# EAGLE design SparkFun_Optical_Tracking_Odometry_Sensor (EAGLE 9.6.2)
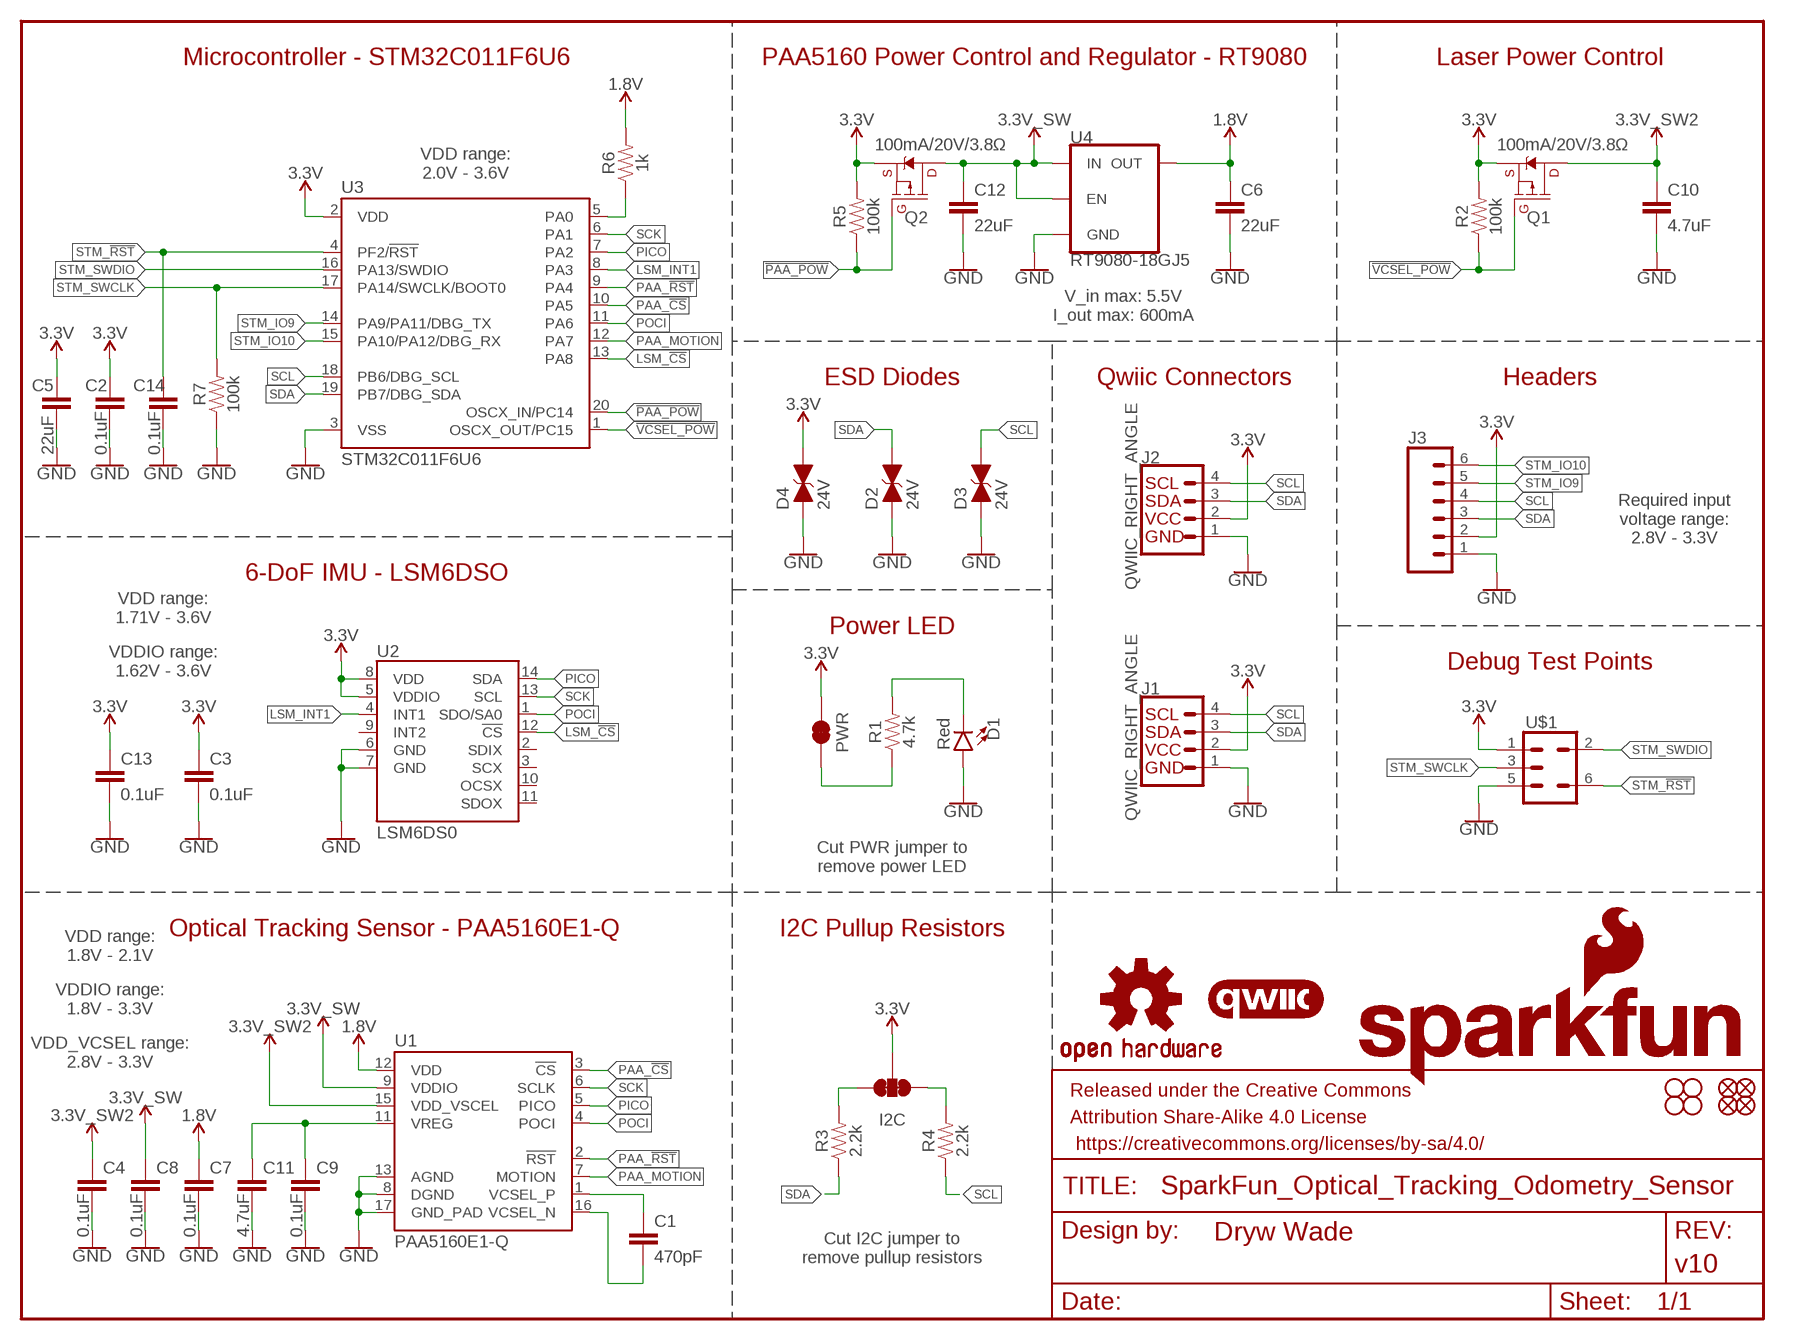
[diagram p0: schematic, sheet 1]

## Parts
C1  470pF  470PF-0603-50V-5%  [0603]
C2  0.1uF  0.1UF-0603-25V-(+80/-20%)  [0603]
C3  0.1uF  0.1UF-0603-25V-(+80/-20%)  [0603]
C4  0.1uF  0.1UF-0603-25V-(+80/-20%)  [0603]
C5  22uF  22UF-0603-6.3V-20%  [0603]
C6  22uF  22UF-0603-6.3V-20%  [0603]
C7  0.1uF  0.1UF-0603-25V-(+80/-20%)  [0603]
C8  0.1uF  0.1UF-0603-25V-(+80/-20%)  [0603]
C9  0.1uF  0.1UF-0603-25V-(+80/-20%)  [0603]
C10  4.7uF  4.7UF-0603-6.3V-(10%)  [0603]
C11  4.7uF  4.7UF-0603-6.3V-(10%)  [0603]
C12  22uF  22UF-0603-6.3V-20%  [0603]
C13  0.1uF  0.1UF-0603-25V-(+80/-20%)  [0603]
C14  0.1uF  0.1UF-0603-25V-(+80/-20%)  [0603]
D1  Red  LED-RED_0603-KB  [LED-0603]
D2  24V  DIODE_TVS  [0603]
D3  24V  DIODE_TVS  [0603]
D4  24V  DIODE_TVS  [0603]
FD1  FIDUCIAL1X2  [FIDUCIAL-1X2]
FD2  FIDUCIAL1X2  [FIDUCIAL-1X2]
FD3  FIDUCIAL1X2  [FIDUCIAL-1X2]
FD4  FIDUCIAL1X2  [FIDUCIAL-1X2]
FRAME1  FRAME-LETTER  [CREATIVE_COMMONS]
H1  STAND-OFF  [STAND-OFF]
H2  STAND-OFF  [STAND-OFF]
H3  STAND-OFF  [STAND-OFF]
H4  STAND-OFF  [STAND-OFF]
I2C  JUMPER-SMT_3_2-NC_TRACE_SILK  [SMT-JUMPER_3_2-NC_TRACE_SILK]
J1  QWIIC_RIGHT_ANGLE  QWIIC_CONNECTORJS-1MM  [JST04_1MM_RA]
J2  QWIIC_RIGHT_ANGLE  QWIIC_CONNECTORJS-1MM  [JST04_1MM_RA]
J3  CONN_06NO_SILK_NO_POP  [1X06_NO_SILK]
LOGO1  OSHW-LOGOS  [OSHW-LOGO-S]
LOGO2  QWIIC_LOGO_5MM  [QWIIC_5MM]
LOGO3  SFE_LOGO_NAME_FLAME.1_INCH  [SFE_LOGO_NAME_FLAME_.1]
PWR  JUMPER-SMT_2_NC_TRACE_SILK  [SMT-JUMPER_2_NC_TRACE_SILK]
Q1  100mA/20V/3.8Ω  MOSFET_PCH-RE1C001ZPTL  [SOT-416FL]
Q2  100mA/20V/3.8Ω  MOSFET_PCH-RE1C001ZPTL  [SOT-416FL]
R1  4.7k  4.7KOHM-0603-1/10W-1%  [0603]
R2  100k  100KOHM-0603-1/10W-1%  [0603]
R3  2.2k  2.2KOHM-0603-1/10W-1%  [0603]
R4  2.2k  2.2KOHM-0603-1/10W-1%  [0603]
R5  100k  100KOHM-0603-1/10W-1%  [0603]
R6  1k  1KOHM-0603-1/10W-1%  [0603]
R7  100k  100KOHM-0603-1/10W-1%  [0603]
U1  PAA5160E1-Q  [PAA5160E1-Q]
U2  LSM6DS0  LSM6DSO  [LGA14L]
U3  STM32C011F6U6  [STM32C011F6U6]
U4  RT9080-18GJ5  V_REG_RT9080-18GJ5  [SOT23-5]
U$1  SWD-5PIN  [PAD_05_03X2_TP_NO4]

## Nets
1.8V: C6.1 C7.1 R6.2 U1.12(VDD) U4.5(OUT)
3.3V: C2.1 C3.1 C5.1 C13.1 D4.2(C) I2C.2 J1.2 J2.2 J3.2 PWR.2 Q1.2(S) Q2.2(S) R2.2 R5.2 U2.5(VDDIO) U2.8(VDD) U3.2(VDD) U$1.1
3.3V_SW: C8.1 C12.1 Q2.3(D) U1.9(VDDIO) U4.1(IN) U4.3(EN)
3.3V_SW2: C4.1 C10.1 Q1.3(D) U1.15(VDD_VSCEL)
!PAA_POW!: Q2.1(G) R5.1 U3.20(OSCX_IN/PC14)
!VCSEL_POW!: Q1.1(G) R2.1 U3.1(OSCX_OUT/PC15)
GND: C2.2 C3.2 C4.2 C5.2 C6.2 C7.2 C8.2 C9.2 C10.2 C11.2 C12.2 C13.2 C14.2 D1.A D2.1(A) D3.1(A) D4.1(A) J1.1 J2.1 J3.1 R7.1 U1.8(DGND) U1.13(AGND) U1.17(GND_PAD) U2.6(GND) U2.7(GND) U3.3(VSS) U4.2(GND) U$1.5
LSM_!CS!: U2.12(!CS!) U3.13(PA8)
LSM_INT1: U2.4(INT1) U3.8(PA3)
N$1: PWR.1 R1.1
N$2: D1.C R1.2
N$3: C1.1 U1.1(VCSEL_P)
N$4: C1.2 U1.16(VCSEL_N)
N$5: I2C.3 R3.2
N$6: I2C.1 R4.2
N$7: C9.1 C11.1 U1.11(VREG)
N$8: R6.1 U3.5(PA0)
PAA_!CS!: U1.3(!CS!) U3.10(PA5)
PAA_!RST!: U1.2(!RST!) U3.9(PA4)
PAA_MOTION: U1.7(MOTION) U3.12(PA7)
PICO: U1.5(PICO) U2.14(SDA) U3.7(PA2)
POCI: U1.4(POCI) U2.1(SDO/SA0) U3.11(PA6)
SCK: U1.6(SCLK) U2.13(SCL) U3.6(PA1)
SCL: D3.2(C) J1.4 J2.4 J3.4 R4.1 U3.18(PB6/DBG_SCL)
SDA: D2.2(C) J1.3 J2.3 J3.3 R3.1 U3.19(PB7/DBG_SDA)
STM_!RST!: C14.1 U3.4(PF2/!RST!) U$1.6
STM_IO9: J3.5 U3.14(PA9/PA11/DBG_TX)
STM_IO10: J3.6 U3.15(PA10/PA12/DBG_RX)
STM_SWCLK: R7.2 U3.17(PA14/SWCLK/BOOT0) U$1.3
STM_SWDIO: U3.16(PA13/SWDIO) U$1.2
Unconnected: U2.2(SDIX) U2.3(SCX) U2.9(INT2) U2.10(OCSX) U2.11(SDOX)

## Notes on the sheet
- Microcontroller - STM32C011F6U6 | PAA5160 Power Control and Regulator - RT9080 | Laser Power Control
- VDD range:
  2.0V - 3.6V
- V_in max: 5.5V
  I_out max: 600mA
- ESD Diodes | Qwiic Connectors | Headers
- Required input
  voltage range:
  2.8V - 3.3V
- 6-DoF IMU - LSM6DSO
- VDD range:
  1.71V - 3.6V
- Power LED
- VDDIO range:
  1.62V - 3.6V
- Debug Test Points
- Cut PWR jumper to
  remove power LED
- Optical Tracking Sensor - PAA5160E1-Q | I2C Pullup Resistors
- VDD range:
  1.8V - 2.1V
- VDDIO range:
  1.8V - 3.3V
- VDD_VCSEL range:
  2.8V - 3.3V
- Cut I2C jumper to
  remove pullup resistors

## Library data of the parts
C1 = SparkFun-Capacitors:470PF: 470pF ceramic capacitors; PROD_ID: CAP-07884
C2-C4 C7-C9 C13 C14 = SparkFun-Capacitors:0.1UF: 0.1µF ceramic capacitors; PROD_ID: CAP-00810
C5 C6 C12 = SparkFun-Capacitors:22UF: 22µF ceramic capacitors; PROD_ID: CAP-14464
C10 C11 = SparkFun-Capacitors:4.7UF: 4.7µF ceramic capacitors; PROD_ID: CAP-08280
D1 = SparkFun-LED:LED-RED: Red SMD LED; PROD_ID: DIO-17976
D2-D4 = SparkFun-DiscreteSemi:DIODE_TVS; PROD_ID: DIO-14502
FD1-FD4 = SparkFun-Aesthetics:FIDUCIAL: Fiducial Alignment Points
FRAME1 = SparkFun-Aesthetics:FRAME-LETTER: Schematic Frame - Letter; DESIGNER: Dryw Wade; REV: v10
H1-H4 = SparkFun-Hardware:STAND-OFF: Stand Off
I2C = SparkFun-Jumpers:JUMPER-SMT_3_2-NC_TRACE: Normally closed trace jumper (2 of 2 connections) This jumper has a trace between all three pads so they are normally closed (NC). Use a razor knife to open the connection(s). For best results follow the IPC guidelines for cutting traces: Cutout at least 0.063 mm (0.005 in). Remove all loose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
J1 J2 = SparkFun-Connectors:QWIIC_CONNECTOR: SparkFun I2C Standard Qwiic Connector An SMD 1mm pitch JST connector makes it easy and quick (get it? Qwiic?) to connect I2C devices to each other. The Qwiic system enables fast and solderless connection between popular platforms and various sensors and actuators. We carry 200mm, 100mm, 50mm, and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; PROD_ID: CONN-13694
J3 = SparkFun-Connectors:CONN_06: Multi connection point. Often used as Generic Header-pin footprint for 0.1 inch spaced/style header connections On any of the 0.1 inch spaced packages, you can populate with these: Break Away Headers - Straight (PRT-00116) Break Away Male Headers - Right Angle (PRT-00553) Female Headers (PRT-00115)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
LOGO1 = SparkFun-Aesthetics:OSHW-LOGO: Open-Source Hardware (OSHW) Logo
LOGO2 = SparkFun-Aesthetics:QWIIC_LOGO: Qwiic Logos for placement on schematic and PCB. The 5.5mm silk logo is best for placing next to Qwiic connector.
LOGO3 = SparkFun-Aesthetics:SFE_LOGO_NAME_FLAME: SparkFun Font Logo w/ Flame
PWR = SparkFun-Jumpers:JUMPER-SMT_2_NC_TRACE: Normally closed trace jumper
Q1 Q2 = SparkFun-DiscreteSemi:MOSFET_PCH: P-channel MOSFETs Voltage controlled devices that allow control of high current outputs. SparkFun Products: SparkFun ESP32 Thing SparkFun ESP8266 Thing SparkFun Pi Servo HAT V2 DMG2305UX-7 (20V/4.2A/SOT23-3); PROD_ID: TRANS-15421
R1 = SparkFun-Resistors:4.7KOHM: 4.7kΩ resistor; PROD_ID: RES-07857
R2 R5 R7 = SparkFun-Resistors:100KOHM: 100kΩ resistor; PROD_ID: RES-07828
R3 R4 = SparkFun-Resistors:2.2KOHM: 2.2kΩ resistor; PROD_ID: RES-08272
R6 = SparkFun-Resistors:1KOHM: 1kΩ resistor; PROD_ID: RES-07856
U1 = Optical_Tracking_Odometry_Sensor:PAA5160E1-Q; PROD_ID: IC-21320
U2 = SparkFun-Sensors:LSM6DSO: The LSM6DSO is a system-in-package featuring a high-performance 3-axis digital accelerometer and 3-axis digital gyroscope.; PROD_ID: IC-15837
U3 = Optical_Tracking_Odometry_Sensor:STM32C011F6U6; PROD_ID: IC-21321
U4 = SparkFun-IC-Power:V_REG_RT9080-18GJ5: RT9080-18GJ5 Low-Dropout Linear Regulator The RT9080 is a low-dropout (LDO) voltage regulators with enable function that operates from 1.2V to 5.5V. It provides up to 600mA of output current and offers low-power operation in miniaturized packaging. The features of low quiescent current as low as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; PROD_ID: VREG-21045
U$1 = SparkFun-Connectors:SWD-5PIN: 5-pin SWD connector Test-point based header for SWD. Pin 1 - PWR Pin 2 - SWDIO Pin 3 - SWCLK Pin 4 - NC Pin 5 - GND Pin 6 - RESET

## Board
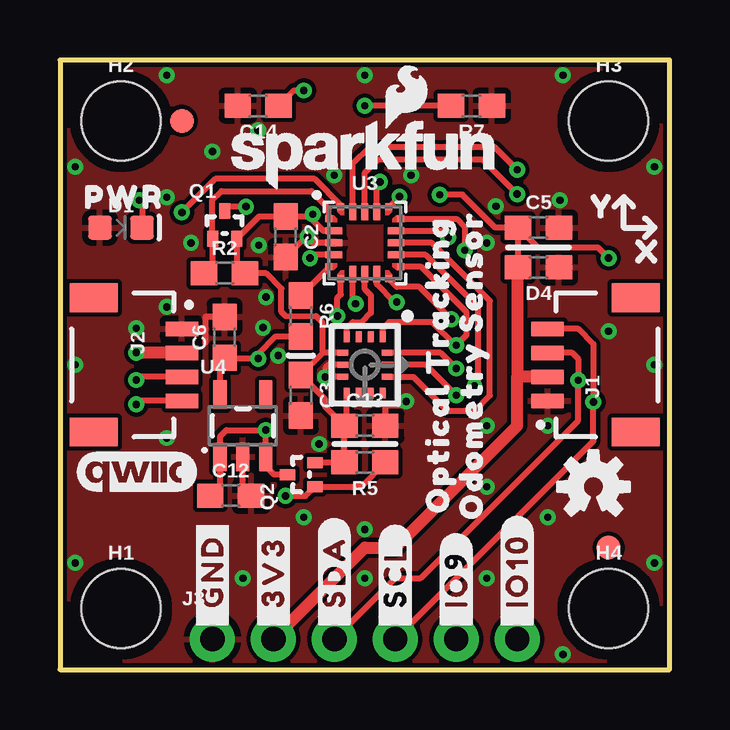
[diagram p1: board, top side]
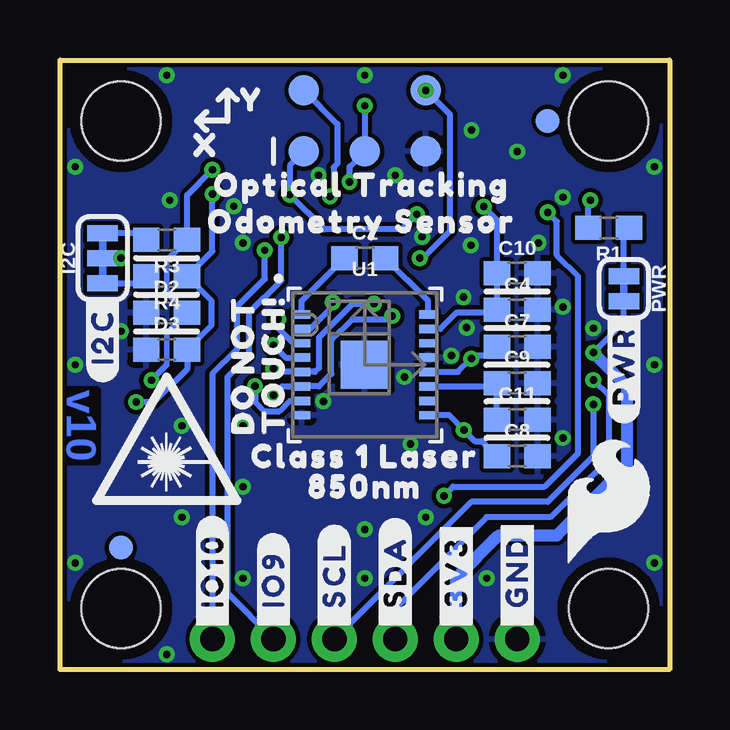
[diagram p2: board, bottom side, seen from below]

Size 25.4 x 25.4 mm. Coordinates in mm from the lower left corner, seen from the top.
Outline: 0,0 25.4,0 25.4,25.4 0,25.4 0,0
Copper layers (1*16): Top 0.035mm / dielectric 1.5mm / Bottom 0.035mm
Design rules "SparkFun-2-Layer-General-JLCPCB": minimum track width 7mil, minimum drill 0.3mm, track to track 7mil, track to pad 7mil, pad to pad 7mil, via to via 7mil, smd to smd 7mil, copper to edge 7mil, drill to drill 7mil, minimum pad ring 7mil, minimum via ring 7mil, stop-mask expansion 3mil, vias tented up to drill 25mil, thermal gap 10mil
tRestrict: area 6.7,16.1 to 7,16.3

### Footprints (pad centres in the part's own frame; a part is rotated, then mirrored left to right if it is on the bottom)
0603 = smd 1.1 x 1: 1 -0.85,0; 2 0.85,0
LED-0603 = smd 1 x 1: A -0.877,0; C 0.877,0
FIDUCIAL-1X2 = smd 1 x 1: 1 0,0
STAND-OFF = hole 3.302: 0,0
SMT-JUMPER_3_2-NC_TRACE_SILK = smd 0.66 x 1.27: 1 -1.041,0; 2 0,0; 3 1.041,0
JST04_1MM_RA = smd 0.6 x 1.35: 1 -1.5,0; 2 -0.5,0; 3 0.5,0; 4 1.5,0 | smd 1.2 x 2: NC1 2.8,-3.675; NC2 -2.8,-3.675
1X06_NO_SILK = drill 1.016 pad 1.88: 1 0,0; 2 2.54,0; 3 5.08,0; 4 7.62,0; 5 10.16,0; 6 12.7,0
SMT-JUMPER_2_NC_TRACE_SILK = smd 0.66 x 1.27: 1 -0.521,0; 2 0.521,0
SOT-416FL = smd 0.46 x 0.65: 1 -0.5,-1.1; 2 0.5,-1.1; 3 0,0.05
PAA5160E1-Q = smd 0.73 x 0.35: 1 -2.635,2.1; 2 -2.635,1.5; 3 -2.635,0.9; 4 -2.635,0.3; 5 -2.635,-0.3; 6 -2.635,-0.9; 7 -2.635,-1.5; 8 -2.635,-2.1; 9 2.635,-2.1; 10 2.635,-1.5; 11 2.635,-0.9; 12 2.635,-0.3; 13 2.635,0.3; 14 2.635,0.9; 15 2.635,1.5; 16 2.635,2.1 | smd 2 x 2: 17 0,0
LGA14L = smd 0.45 x 0.25: 1 -1.175,0.75; 2 -1.175,0.25; 3 -1.175,-0.25; 4 -1.175,-0.75; 8 1.175,-0.75; 9 1.175,-0.25; 10 1.175,0.25; 11 1.175,0.75 | smd 0.25 x 0.45: 5 -0.5,-0.925; 6 0,-0.925; 7 0.5,-0.925; 12 0.5,0.925; 13 0,0.925; 14 -0.5,0.925
STM32C011F6U6 = smd 0.3 x 0.3: 1 -1.5,1; 5 -1.5,-1; 6 -1,-1.5; 10 1,-1.5; 11 1.5,-1; 15 1.5,1; 16 1,1.5; 20 -1,1.5 | smd 0.7 x 0.3: 2 -1.3,0.5; 3 -1.3,0; 4 -1.3,-0.5; 12 1.3,-0.5; 13 1.3,0; 14 1.3,0.5 | smd 0.3 x 0.7: 7 -0.5,-1.3; 8 0,-1.3; 9 0.5,-1.3; 17 0.5,1.3; 18 0,1.3; 19 -0.5,1.3
SOT23-5 = smd 0.55 x 1.2: 1 -0.95,-1.3; 2 0,-1.3; 3 0.95,-1.3; 4 0.95,1.3; 5 -0.95,1.3
PAD_05_03X2_TP_NO4 = smd 1.27 x 1.27: 1 -2.54,-1.27; 2 -2.54,1.27; 3 0,-1.27; 5 2.54,-1.27; 6 2.54,1.27

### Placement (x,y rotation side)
C1  12.7,17.14 0 bottom
C2  9.4,18.03 270 top
C3  10.03,11.43 270 top
C4  6.35,14.99 0 bottom
C5  19.94,18.41 0 top
C6  6.86,13.84 90 top
C7  6.35,13.46 0 bottom
C8  6.35,8.89 0 bottom
C9  6.35,11.94 0 bottom
C10  6.35,16.51 0 bottom
C11  6.35,10.41 0 bottom
C12  7.11,7.24 0 top
C13  12.7,10.16 0 top
C14  8.26,23.5 180 top
D1  2.54,18.41 0 top
D2  20.95,14.86 0 bottom
D3  20.95,13.34 0 bottom
D4  19.94,16.76 180 top
FD1  5.08,22.86 0 bottom
FD2  5.08,22.86 0 top
FD3  22.86,5.08 0 bottom
FD4  22.86,5.08 0 top
FRAME1  not placed on the board
H1  2.54,2.54 0 top
H2  2.54,22.86 0 top
H3  22.86,22.86 0 top
H4  22.86,2.54 0 top
I2C  23.62,17.14 90 bottom
J1  20.32,12.7 90 top
J2  5.08,12.7 270 top
J3  6.35,1.27 0 top
LOGO1  22.23,7.62 0 top
LOGO2  3.17,8.26 0 top
LOGO3  12.7,21.46 0 top
PWR  1.91,15.88 270 bottom
Q1  6.86,19.05 0 top
Q2  9.53,8.13 90 top
R1  2.54,18.41 180 bottom
R2  6.86,16.51 0 top
R3  20.95,17.91 180 bottom
R4  20.95,16.38 180 bottom
R5  12.7,8.64 180 top
R6  10.03,14.73 270 top
R7  17.14,23.5 180 top
U1  12.7,12.7 0 bottom
U2  12.7,12.7 270 top
U3  12.7,17.78 0 top
U4  7.62,10.16 0 top
U$1  12.7,22.86 0 bottom
U$2  [#_GND#0]  6.35,1.52 90 top
U$3  [#_3V3#0]  8.89,1.52 90 top
U$4  [#_SDA#0]  11.43,1.52 90 top
U$5  [#_SCL#0]  13.97,1.52 90 top
U$6  [CLASS_1_LASER0]  12.7,8.89 0 bottom
U$7  [#_IO10#0]  19.05,1.52 90 top
U$8  [#_GND#0]  6.35,1.52 90 bottom
U$9  [#_3V3#0]  8.89,1.52 90 bottom
U$10  [#_SDA#0]  11.43,1.52 90 bottom
U$11  [#_SCL#0]  13.97,1.52 90 bottom
U$12  [#_IO9#0]  16.51,1.52 90 top
U$14  [OPTICAL_TRACKING0]  12.83,20.19 0 bottom
U$15  [ODOMETRY_SENSOR0]  12.83,18.67 0 bottom
U$16  [OPTICAL_TRACKING0]  15.75,12.7 90 top
U$17  [ODOMETRY_SENSOR0]  17.14,12.7 90 top
U$18  [X0]  24.51,17.4 0 top
U$20  [#PWR#0]  1.91,14.99 90 bottom
U$21  [TOUCH##0]  16.51,12.7 90 bottom
U$22  [DO_NOT0]  17.78,12.7 90 bottom
U$23  [#_IO10#0]  19.05,1.52 90 bottom
U$24  [SFE_LOGO_FLAME_.2]  2.54,6.99 0 bottom
U$25  [PWR0]  2.67,19.68 0 top
U$26  [#I2C#0]  23.62,15.75 90 bottom
U$27  [ORDERING_INSTRUCTIONS]  not placed on the board
U$28  [850NM0]  12.7,7.62 0 bottom
U$29  [Y0]  22.61,19.3 0 top
U$30  [X0]  19.3,21.84 0 bottom
U$31  [Y0]  17.4,23.75 0 bottom
U$32  [#_IO9#0]  16.51,1.52 90 bottom

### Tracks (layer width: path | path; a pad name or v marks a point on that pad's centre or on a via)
1.8V  (via drill 0.3)
  Top 0.254: U4.5 6.67,12.8 C6.1 6.89,12.96 v8.26,12.96 8.26,13.15 8.99,13.88 R6.2
  Bottom 0.254: C7.1 7.56,13.11 8.11,13.11 v8.26,12.96 8.82,12.4 U1.12
3.3V  (via drill 0.3)
  Top 0.229: 10.67,14.73 9.4,14.73
  Top 0.254: C13.1 11.95,10.26 U2.8 | 10.94,13.19 C3.1 11.05,11.26 11.05,10.96 C13.1 | 10.94,13.19 10.95,13.2 U2.5 | U3.2 10.97,18.28 10.53,18.72 v10.53,18.97 10.44,18.88 C2.1 8.29,18.88 Q1.2 7.36,16.86 R2.2 8.59,16.51 9.22,15.88 9.22,14.91 9.4,14.73 | 10.94,13.19 10.94,14.45 10.92,14.47 10.92,14.48 10.67,14.73 | Q2.2 10.63,8.64 R5.2 C13.1 | 19.05,16.73 D4.2 C5.1 | v22.86,17.14 22.42,17.59 19.91,17.59 C5.1 | C5.1 18.14,18.41 16.77,19.79 v15.82,19.79
  Top 0.508: J2.2 3.18,13.2 v3.17,13.21 | J3.2 12.7,5.08 13.97,5.08 19.05,10.16 19.05,12.2 | J1.2 19.05,12.2 | 19.05,16.73 19.05,12.2
  Bottom 0.254: v10.53,18.97 11.17,18.34 14.38,18.34 v15.82,19.79 15.82,21.01 U$1.1 | I2C.2 v22.86,17.14 | v3.17,13.21 1.91,14.48 PWR.2
  Bottom 0.508: J3.2 8.89,3.81 7.11,5.59 4.7,5.59 1.78,8.51 1.78,11.81 v3.17,13.21
3.3V_SW  (via drill 0.3)
  Top 0.254: C12.1 6.67,7.65 U4.1 6.67,9.72 6.93,9.98 v8.57,9.98 U4.3 8.57,8.48 8.92,8.13 Q2.3
  Bottom 0.254: C8.1 7.83,9.53 8.12,9.53 v8.57,9.98 9.19,10.6 U1.9
3.3V_SW2  (via drill 0.3)
  Top 0.254: Q1.3 7.05,19.29 v7.75,19.29
  Bottom 0.254: U1.15 9.55,14.2 8.87,14.88 7.3,14.88 C4.1 C10.1 7.2,18.74 v7.75,19.29
!PAA_POW!  (via drill 0.3)
  Top 0.254: U3.20 11.7,19.36 10.61,20.45 6.48,20.45 v5.08,19.05 | R5.1 12.54,7.63 Q2.1 10.24,7.24 v9.4,7.24
  Bottom 0.254: v5.08,19.05 4.7,18.67 4.7,17.27 3.81,16.38 3.81,9.02 5.21,7.62 9.02,7.62 v9.4,7.24
!VCSEL_POW!
  Top 0.254: U3.1 11.2,19.21 10.47,19.94 6.73,19.94 6.32,19.53 6.32,17.98 Q1.1 6.36,16.86 R2.1
GND  (via drill 0.3)
  Top 0.254: U2.7 v11.06,12.2 | v11.06,12.2 v11.05,12.19 | U2.6 11.18,12.7 11.06,12.57 v11.06,12.2 | U3.3 10.51,17.78 10.38,17.91 10.12,17.91 C2.2 | C12.2 7.62,7.58 U4.2 | C6.2 6.05,14.69 6.05,14.22 | 6.05,14.22 6.05,13.63 | J2.1 6.03,14.2 6.05,14.22 | v14.43,11.18 14.25,10.99 13.55,10.99 C13.2
  other vias: 9.09,13.08 4.45,15.11 4.45,9.65 3.17,14.22 8.59,15.52 8.46,14.25 10.79,9.4 5.46,17.78 8.28,17.68 20.32,10.16 17.78,7.62 17.78,10.16 17.78,3.81 20.32,6.35 17.78,17.78 22.86,14.1 18.16,19.3 20.83,19.56 11.43,20.6 4.45,19.68 14.63,20.6 10.16,6.35 20.95,24.77 24.77,20.95 20.95,0.64 24.77,4.45 0.64,4.45 24.77,12.7 0.64,12.7 0.64,20.95 4.45,24.77 12.7,24.77 12.7,3.81 12.7,5.84 10.31,18.03 7.62,3.81 8.26,22.48 6.35,21.59
  pour Top (isolate 0.178): 0,0 25.4,0 25.4,25.4 0,25.4
  pour Bottom (isolate 0.178): 25.4,0 0,0 0,25.4 25.4,25.4
LSM_!CS!
  Top 0.254: U2.12 14.72,12.2 16.13,10.79 17.27,10.79 17.91,11.43 17.91,15.37 15.49,17.78 U3.13
LSM_INT1
  Top 0.254: U2.4 11.95,14.22 12.2,14.48 12.57,14.48 12.95,14.86 12.95,15.59 12.7,15.85 U3.8
N$1
  Bottom 0.254: PWR.1 1.91,18.2 R1.1
N$2  (via drill 0.3)
  Top 0.254: v3.3,19.56 3.42,19.44 D1.C
  Bottom 0.254: R1.2 3.39,19.47 v3.3,19.56
N$3
  Bottom 0.254: U1.1 15.34,15.36 C1.1
N$4
  Bottom 0.254: U1.16 10.06,15.36 C1.2
N$5
  Bottom 0.254: R3.2 22.08,18.19 I2C.3
N$6
  Bottom 0.254: I2C.1 22.08,16.1 R4.2
N$7
  Bottom 0.254: U1.11 7.34,11.8 C9.1 C11.1
N$8
  Top 0.254: U3.5 11.2,16.75 R6.1
PAA_!CS!  (via drill 0.3)
  Top 0.254: v16.31,14.61 14.96,15.95 14.03,15.95 U3.10
  Bottom 0.254: v16.31,14.61 16.31,14.22 15.68,13.6 U1.3
PAA_!RST!  (via drill 0.3)
  Top 0.254: v14.03,15.31 13.94,15.31 13.2,16.05 U3.9
  Bottom 0.254: U1.2 14.96,14.2 14.03,15.13 v14.03,15.31
PAA_MOTION  (via drill 0.3)
  Top 0.254: v17.27,11.81 17.4,11.94 17.4,15.11 15.23,17.28 U3.12
  Bottom 0.254: v17.27,11.81 17.27,11.15 16.89,10.77 16.25,10.77 15.82,11.2 U1.7
PICO  (via drill 0.3)
  Top 0.254: v12.32,15.24 12.2,15.36 U3.7 | v16.51,12.55 15.86,13.2 U2.14
  Bottom 0.254: v12.32,15.24 13.21,15.24 14.61,13.84 14.61,12.57 14.78,12.4 U1.5 16.36,12.4 v16.51,12.55
POCI  (via drill 0.3)
  Top 0.254: U2.1 13.45,14.21 13.72,14.48 15.52,14.48 16.48,13.51 v16.51,13.51 16.94,13.95 16.94,14.88 15.05,16.78 U3.11
  Bottom 0.254: v16.51,13.51 16,13 U1.4
SCK  (via drill 0.3)
  Top 0.254: v16.51,11.43 15.24,12.7 U2.13 | v11.56,14.73 11.56,15.49 11.7,15.64 U3.6
  Bottom 0.254: v16.51,11.43 16.14,11.8 U1.6 14.62,11.8 14.1,12.32 14.1,13.72 13.21,14.61 11.68,14.61 v11.56,14.73
SCL  (via drill 0.3)
  Top 0.254: U3.18 12.7,20.7 13.23,21.23 17.62,21.23 v19.05,19.81 | J2.4 3.33,11.2 v3.17,11.05 | J1.4 21.59,14.2 22.23,13.56 v22.23,11.15 22.23,9.53 J3.4
  Bottom 0.254: v3.17,11.05 3.17,8.89 5.08,6.99 8.26,6.99 J3.4 | v22.23,11.15 21.46,11.15 20.11,12.51 D3.2 19.09,14.35 19.09,15.37 R4.1 19.05,17.44 v19.05,19.81
SDA  (via drill 0.3)
  Top 0.254: U3.19 12.2,21.09 12.88,21.77 18.11,21.77 v19.05,20.83 | J2.3 3.31,12.2 v3.17,12.06 | J3.3 13.97,3.81 15.03,3.81 21.59,10.38 v21.59,12.06 21.59,12.95 21.34,13.2 J1.3
  Bottom 0.229: 20.95,14.01 20.95,12.69 v21.59,12.06 | 20.95,17.06 20.95,15.71
  Bottom 0.254: v3.17,12.06 2.54,11.43 2.54,8.76 4.95,6.35 7.62,6.35 11.43,2.54 J3.3 | 20.95,14.01 D2.2 20.95,15.71 | 20.95,17.06 R3.1 20.11,19.77 v19.05,20.83
STM_!RST!  (via drill 0.3)
  Top 0.254: U3.4 10.55,17.28 v10.41,17.14 | U$1.6 9.74,24.13 C14.1
  Bottom 0.254: v10.41,17.14 10.29,17.14 9.14,18.29 9.14,23.11 U$1.6
  other vias: 10.16,24.13
STM_IO9  (via drill 0.3)
  Top 0.254: U3.14 15.86,18.28 16.13,18.01 v16.18,18.01
  Bottom 0.254: v16.18,18.01 16.18,16.2 17.53,14.86 17.53,13.08 18.41,12.19 18.41,3.17 J3.5
STM_IO10  (via drill 0.3)
  Top 0.254: U3.15 16.53,18.78 16.87,18.44 v16.87,17.48
  Bottom 0.254: v16.87,17.48 16.87,16.28 18.03,15.11 18.03,13.34 19.05,12.32 J3.6
STM_SWCLK  (via drill 0.3)
  Top 0.254: U3.17 13.2,20.18 v13.34,20.32 | R7.2 v12.7,23.5
  Bottom 0.254: v13.34,20.32 13.34,20.95 U$1.3 v12.7,23.5
STM_SWDIO  (via drill 0.3)
  Top 0.254: U3.16 13.72,19.28 v14.15,19.71
  Bottom 0.254: v14.15,19.71 13.99,19.86 13.99,20.93 13.84,21.08 13.84,22.73 U$1.2

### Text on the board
Bottom: v10
Measures: Units: inches
tDocu: 2-layer / 1oz copper / Board thickness: 1.6mm / Material: TG135-140 / Soldermask: Red / Silkscreen: White / Surface Finish: Lead-Free HASL | Dryw Wade

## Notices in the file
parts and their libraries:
SparkFun-Aesthetics: Licensing: Creative Commons ShareAlike 4.0 International - https://creativecommons.org/licenses/by-sa/4.0
SparkFun-Aesthetics: Released under the Creative Commons Attribution Share-Alike 4.0 License
SparkFun-Aesthetics: https://creativecommons.org/licenses/by-sa/4.0
